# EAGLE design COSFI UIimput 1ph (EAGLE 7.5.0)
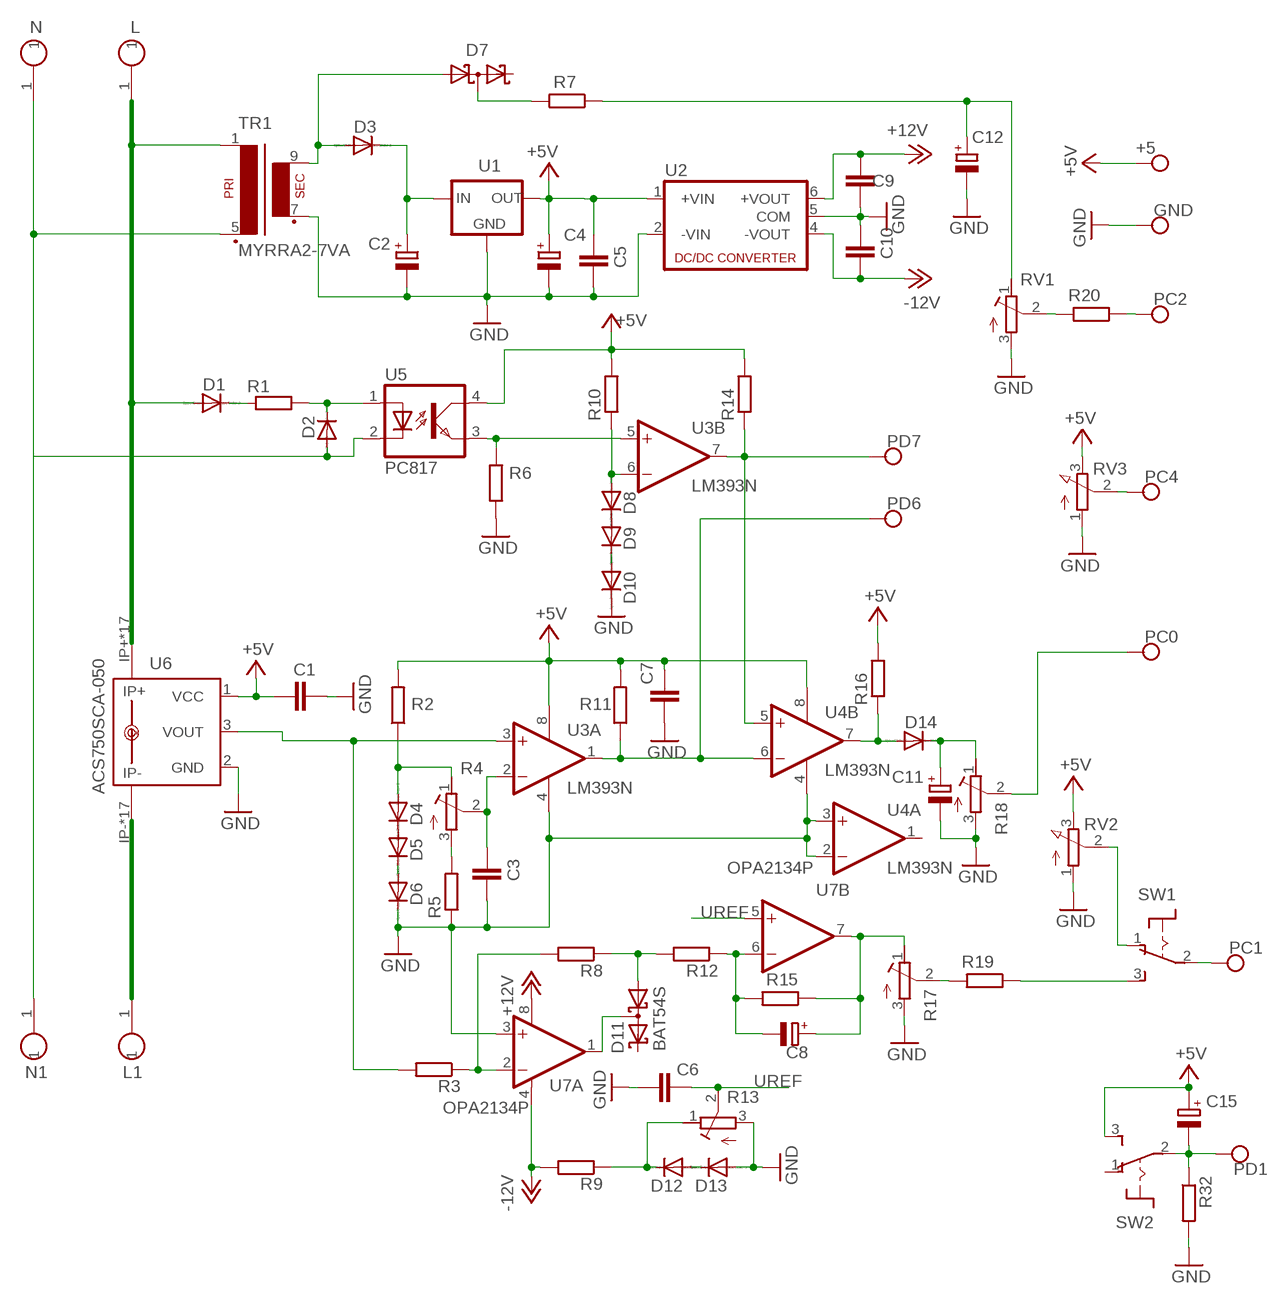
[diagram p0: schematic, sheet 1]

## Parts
+5  CONNWIRE  [CONNWIRE]
C1  C-EUC1206  [C1206]
C2  CPOL-EUE5-8.5  [E5-8,5]
C3  C-EUC1206  [C1206]
C4  CPOL-EUE2-5  [E2-5]
C5  C-EUC1206  [C1206]
C6  C-EUC1206  [C1206]
C7  C-EUC1206  [C1206]
C8  CPOL-EUE2-5  [E2-5]
C9  C-EUC1206  [C1206]
C10  C-EUC1206  [C1206]
C11  CPOL-EUE2-5  [E2-5]
C12  CPOL-EUE3.5-8  [E3,5-8]
C15  CPOL-EUE2-5  [E2-5]
D1  1N4004  [DO41-10]
D2  1N4004  [DO41-10]
D3  1N4004  [DO41-10]
D4  1N4148DO35-7  [DO35-7]
D5  1N4148DO35-7  [DO35-7]
D6  1N4148DO35-7  [DO35-7]
D7  BAT54S  [SOT23]
D8  1N4148DO35-7  [DO35-7]
D9  1N4148DO35-7  [DO35-7]
D10  1N4148DO35-7  [DO35-7]
D11  BAT54S  [SOT23]
D12  1N4148DO35-7  [DO35-7]
D13  1N4148DO35-7  [DO35-7]
D14  1N4148DO35-7  [DO35-7]
GND  CONNWIRE  [CONNWIRE]
L  CONNHOLE  [CONNHOLE4]
L1  CONNHOLE  [CONNHOLE4]
N  CONNHOLE  [CONNHOLE4]
N1  CONNHOLE  [CONNHOLE4]
PC0  CONNWIRE  [CONNWIRE]
PC1  CONNWIRE  [CONNWIRE]
PC2  CONNWIRE  [CONNWIRE]
PC4  CONNWIRE  [CONNWIRE]
PD1  CONNWIRE  [CONNWIRE]
PD6  CONNWIRE  [CONNWIRE]
PD7  CONNWIRE  [CONNWIRE]
R1  R-EU_0617/22  [0617/22]
R2  R-EU_0204/7  [0204/7]
R3  R-EU_0204/7  [0204/7]
R4  R-TRIMM-3386-F  [R-TRIMM-3386F]
R5  R-EU_0204/7  [0204/7]
R6  R-EU_0204/7  [0204/7]
R7  R-EU_0204/7  [0204/7]
R8  R-EU_0204/7  [0204/7]
R9  R-EU_0204/7  [0204/7]
R10  R-EU_0204/7  [0204/7]
R11  R-EU_0204/7  [0204/7]
R12  R-EU_0204/7  [0204/7]
R13  R-TRIMM-3386-F  [R-TRIMM-3386F]
R14  R-EU_0204/7  [0204/7]
R15  R-EU_0204/7  [0204/7]
R16  R-EU_0204/7  [0204/7]
R17  R-TRIMM-3386-F  [R-TRIMM-3386F]
R18  R-TRIMM-3386-F  [R-TRIMM-3386F]
R19  R-EU_0204/7  [0204/7]
R20  R-EU_0204/7  [0204/7]
R32  R-EU_0204/7  [0204/7]
RV1  R-TRIMM-3386-F  [R-TRIMM-3386F]
RV2  PTV09A  PV09A  [PTV09]
RV3  PTV09A  PV09A  [PTV09]
SW1  8MS9P1  [8MS9]
SW2  8MS9P1  [8MS9]
TR1  MYRRA2-7VA  [MYRRA2-7]
U1  78XXL  [78XXL]
U2  NMA  [NMA]
U3  LM393N  [DIL08]
U4  LM393N  [DIL08]
U5  PC817  [DIL04]
U6  ACS750SCA-050  [ACS75050]
U7  OPA2134P  [DIL08]

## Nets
+5V: +5.P$1 C1.2 C4.+ C5.1 C7.2 C15.+ R2.2 R10.2 R11.2 R14.2 R16.2 RV2.3(E) RV3.3(E) SW2.3(S) U1.OUT U2.1(+VIN) U3.8(P:V+) U4.8(P:V+) U5.4(COL) U6.1(VCC)
+12V: C9.1 U2.6(+VOUT) U7.8(A:V+)
-12V: C10.2 R9.2 U2.4(-VOUT) U7.4(A:V-)
GND: C1.1 C2.- C3.2 C4.- C5.2 C6.1 C7.1 C9.2 C10.1 C11.- C12.- D6.C D10.C D13.A GND.P$1 R5.1 R6.1 R13.3(E) R17.3(E) R18.3(E) R32.2 RV1.3(E) RV2.1(A) RV3.1(A) TR1.7(S3) U1.GND U2.2(-VIN) U2.5(COM) U3.4(P:V-) U4.2(A:-IN) U4.3(A:+IN) U4.4(P:V-) U6.2(GND) U7.3(A:+IN)
N$1: D1.C R1.1
N$2: R3.1 R8.2 U7.2(A:-IN)
N$3: D2.C R1.2 U5.1(A)
N$4: D8.C D9.A
N$5: D2.A N1.1 N.1 TR1.5(P2) U5.2(C)
N$6: D1.A L.1 TR1.1 U6.IP+ U6.IP+@2(IP+) U6.IP+@3(IP+) U6.IP+@4(IP+) U6.IP+@5(IP+) U6.IP+@6(IP+) U6.IP+@7(IP+) U6.IP+@8(IP+) U6.IP+@9(IP+) U6.IP+@10(IP+) U6.IP+@11(IP+) U6.IP+@12(IP+) U6.IP+@13(IP+) U6.IP+@14(IP+) U6.IP+@15(IP+) U6.IP+@16(IP+) U6.IP+@17(IP+)
N$7: RV2.2(S) SW1.1(O)
N$8: D9.C D10.A
N$9: D12.A D13.C
N$10: D12.C R9.1 R13.1(A)
N$11: R4.3(E) R5.2
N$12: D4.A R2.1 R4.1(A)
N$13: R6.2 U3.5(B:+IN) U5.3(EMIT)
N$14: R3.2 U3.3(A:+IN) U6.3(VOUT)
N$15: D4.C D5.A
N$16: D8.A R10.1 U3.6(B:-IN)
N$17: D14.A R16.1 U4.7(B:OUT)
N$18: PD7.P$1 R14.1 U3.7(B:OUT) U4.5(B:+IN)
N$19: D5.C D6.A
N$20: PD6.P$1 R11.1 U3.1(A:OUT) U4.6(B:-IN)
N$21: C3.1 R4.2(S) U3.2(A:-IN)
N$22: C11.+ D14.C R18.1(A)
N$23: PC0.P$1 R18.2(S)
N$24: D11.3(C1A2) U7.1(A:OUT)
N$25: PC1.P$1 SW1.2(P)
N$26: PC4.P$1 RV3.2(S)
N$27: R19.1 SW1.3(S)
N$28: PC2.P$1 R20.1
N$29: D3.A D7.1(A1) TR1.9(S4)
N$30: D7.3(C1A2) R7.2
N$31: D11.1(A1) R8.1 R12.2
N$32: C8.- R12.1 R15.2 U7.6(B:-IN)
N$33: C8.+ R15.1 R17.1(A) U7.7(B:OUT)
N$34: C15.- PD1.P$1 R32.1 SW2.2(P)
N$35: R17.2(S) R19.2
N$37: C2.+ D3.C U1.IN
N$38: R20.2 RV1.2(S)
N$40: C12.+ R7.1 RV1.1(A)
N$41: L1.1 U6.IP- U6.IP-@2(IP-) U6.IP-@3(IP-) U6.IP-@4(IP-) U6.IP-@5(IP-) U6.IP-@6(IP-) U6.IP-@7(IP-) U6.IP-@8(IP-) U6.IP-@9(IP-) U6.IP-@10(IP-) U6.IP-@11(IP-) U6.IP-@12(IP-) U6.IP-@13(IP-) U6.IP-@14(IP-) U6.IP-@15(IP-) U6.IP-@16(IP-) U6.IP-@17(IP-)
UREF: C6.2 R13.2(S) U7.5(B:+IN)
Unconnected: D7.2(C2) D11.2(C2) SW2.1(O) U4.1(A:OUT)

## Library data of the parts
+5 GND PC0 PC1 PC2 PC4 PD1 PD6 PD7 = connholes:CONNWIRE
C1 C3 C5-C7 C9 C10 = rcl:C-EU: CAPACITOR, European symbol
C2 C4 C8 C11 C12 C15 = rcl:CPOL-EU: POLARIZED CAPACITOR, European symbol
D1-D3 = diode:1N4004: DIODE
D4-D6 D8-D10 D12-D14 = diode:1N4148: DIODE
D7 D11 = diode:BAT54S: Schottky Diodes Pin connection corrected 2011-05-04 Source: Fairchild .. BAT54.pdf
L L1 N N1 = connholes:CONNHOLE
R1-R3 R5-R12 R14-R16 R19 R20 R32 = rcl:R-EU_: RESISTOR, European symbol
R4 R13 R17 R18 RV1 = rcl:R-TRIMM-3386-F
RV2 RV3 = pot:PV09A
SW1 SW2 = switch:8MS9P1
TR1 = trafo:MYRRA2-7VA
U1 = v-reg:78XXL: VOLTAGE REGULATOR
U2 = dc-dc-converter:NMA: DC-DC CONVERTER; MF: C & D TECHNOLOGIES, INC; MPN: NMA0515SC; OC_FARNELL: 1021434; OC_NEWARK: 61K3064
U3 U4 = linear:LM393: COMPARATOR
U5 = optocoupler:PC817: SHARP OPTO COUPLER; MPN: PC817X4J000F; OC_FARNELL: 9707727; OC_NEWARK: 97K7059
U6 = allegro:ACS750*CA-050: Current Sensor display layer 49 Reference in BRD and place VIAs on circles Source: www.allegromicro.com/datafile/0750-050.pdf; MF: ALLEGRO MICROSYSTEMS, INC.; MPN: ACS750SCA-050; OC_FARNELL: 1457175; OC_NEWARK: 81H6588
U7 = burr-brown:OPA2134: Operational Amplifier; MF: TEXAS INSTRUMENTS; MPN: OPA2134PA; OC_FARNELL: 1097574; OC_NEWARK: 74K3897

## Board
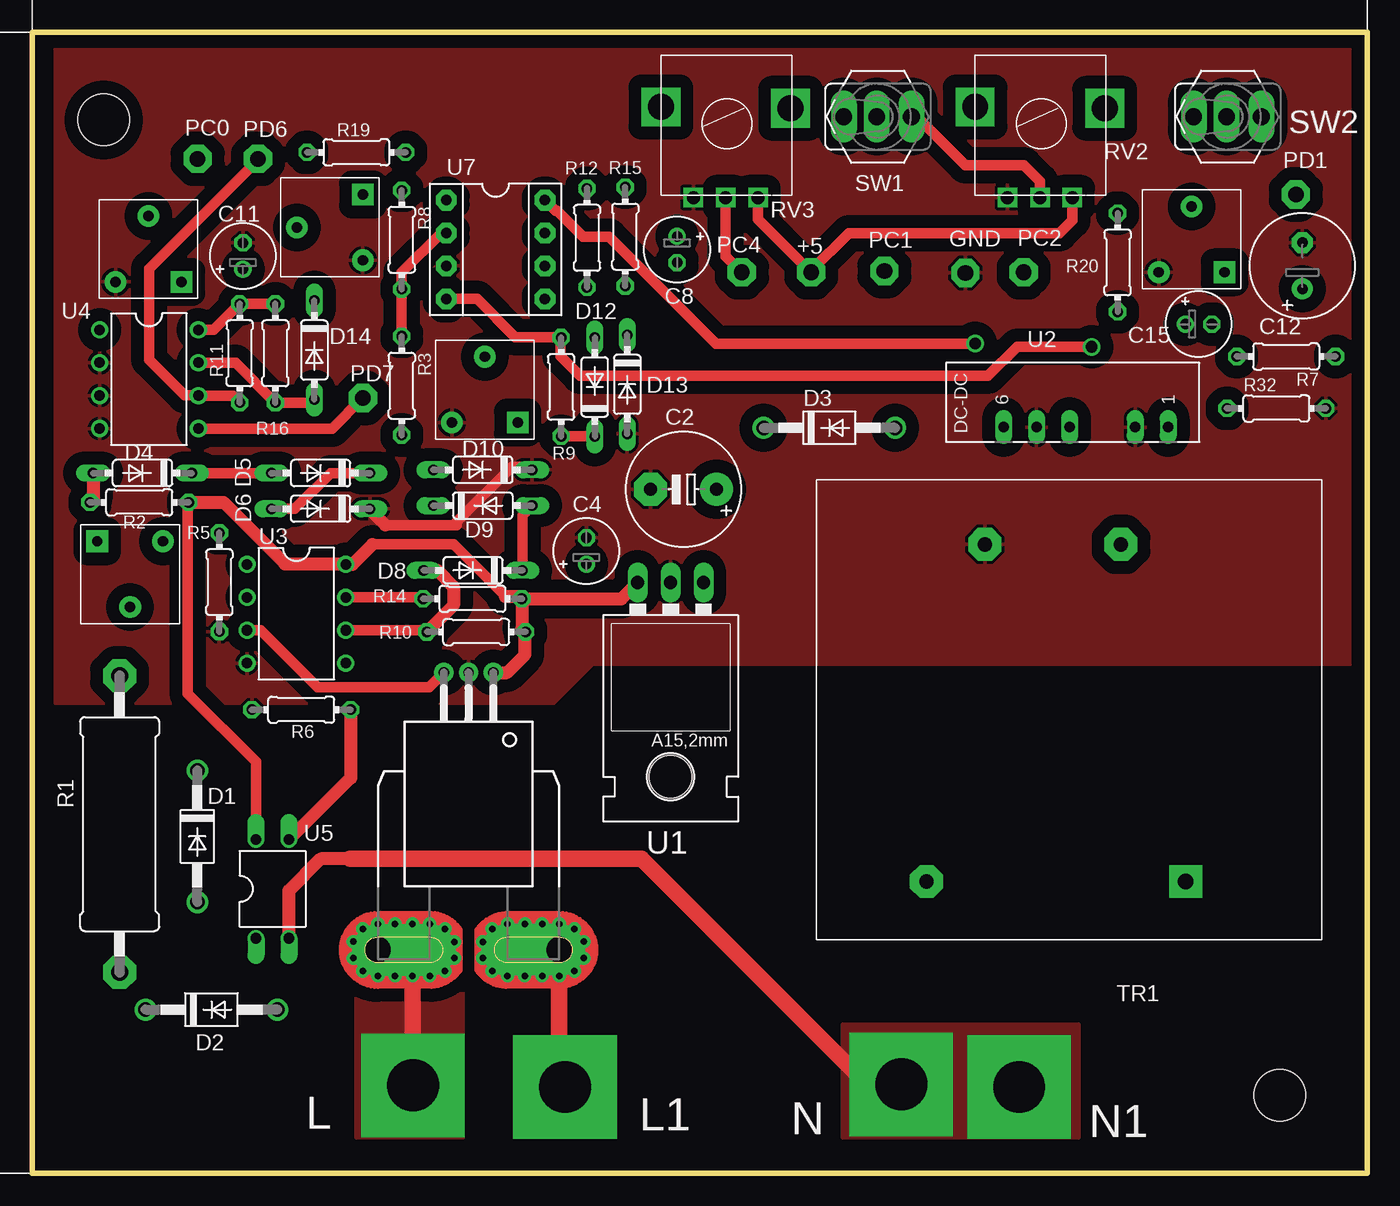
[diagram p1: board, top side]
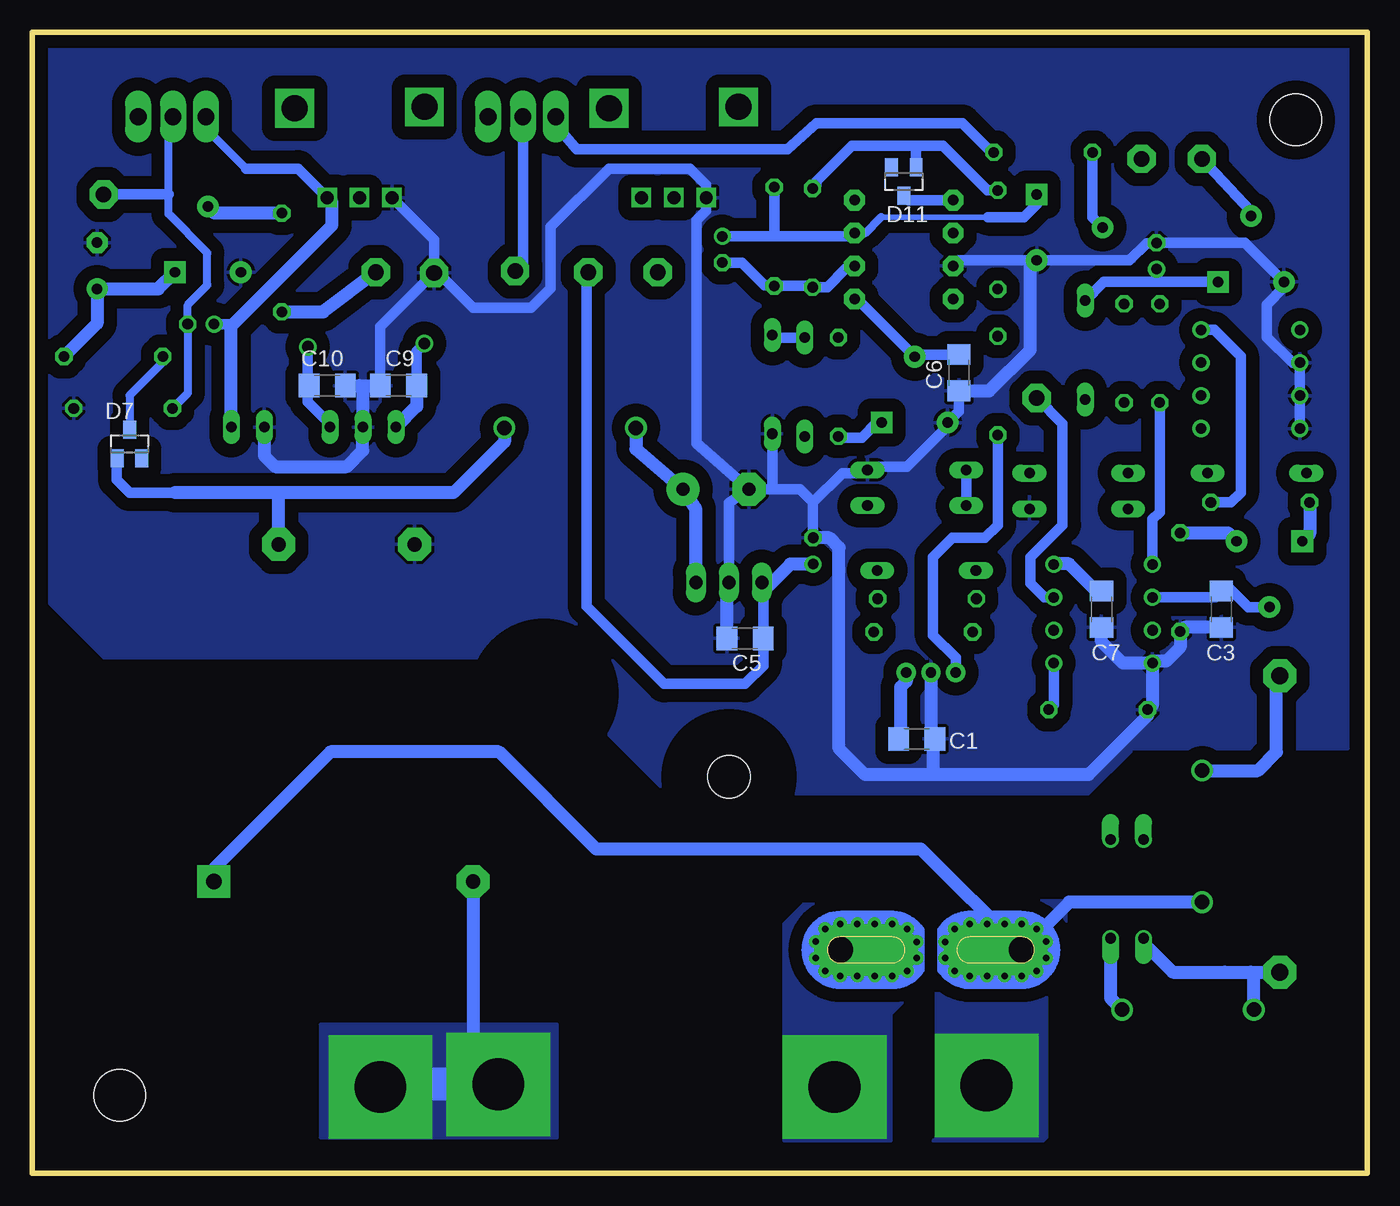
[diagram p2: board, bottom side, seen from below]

Size 103 x 88 mm. Coordinates in mm from the lower left corner, seen from the top.
Outline: 0,0 103,0 103,88 0,88 0,0
Copper layers (1*16): Top 0.035mm / dielectric 1.5mm / Bottom 0.035mm
Design rules "default": minimum track width 10mil, minimum drill 24mil, track to track 8mil, track to pad 8mil, pad to pad 8mil, via to via 8mil, smd to smd 8mil, copper to edge 40mil, drill to drill 8mil, minimum pad ring 10mil, minimum via ring 8mil, stop-mask expansion 4mil, vias tented up to drill 0mil, thermal gap 10mil
Holes 4 mm at 96.25,6 5.5,81.25
bRestrict: area 58.9,32.4 to 68.1,41.6

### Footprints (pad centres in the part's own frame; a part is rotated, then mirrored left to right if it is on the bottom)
CONNWIRE = drill 1.2 pad 2.184 octagon: P$1 0,0
C1206 = smd 1.6 x 1.8: 1 -1.4,0; 2 1.4,0
E5-8,5 = drill 1.016 pad 2.54: + -2.54,0 | drill 1.016 pad 2.54 octagon: - 2.54,0
E2-5 = drill 0.813 pad 1.27: + -1.016,0 | drill 0.813 pad 1.27 octagon: - 1.016,0
E3,5-8 = drill 0.813 pad 1.6: + -1.778,0 | drill 0.813 pad 1.6 octagon: - 1.778,0
DO41-10 = drill 1.118: A 5.08,0; C -5.08,0
DO35-7 = drill 0.813 long: A 3.81,0; C -3.81,0
SOT23 = smd 1 x 1.4: 1 -0.95,-1.1; 2 0.95,-1.1; 3 0,1.1
CONNHOLE4 = drill 4 pad 8 square: 1 0,0
0617/22 = drill 1.3 pad 2.54 octagon: 1 -11.43,0; 2 11.43,0
0204/7 = drill 0.813 octagon: 1 -3.81,0; 2 3.81,0
R-TRIMM-3386F = drill 0.8 pad 1.676 square: 1 0,0 | drill 0.8 pad 1.676: 2 5.08,2.54; 3 0,5.08
PTV09 = drill 1 square: 1 -2.5,0; 2 0,0; 3 2.5,0 | drill 2 square: P$4 -5,7; P$5 5,6.9
8MS9 = drill 1.295 pad 2 long: 1 -3,5.346 | drill 1.3 pad 2 long: 2 -3,2.654; 3 -3,0.114
MYRRA2-7 = drill 1.2 pad 2.54 square: 1 0,0 | drill 1.1 pad 2.54 octagon: 5 20,0; 7 15.5,-26; 9 5,-26
78XXL = drill 1.016 long: GND 0,-3.81; IN -2.54,-3.81; OUT 2.54,-3.81 | hole 3.302: 0,11.176
NMA = drill 0.813 long: 1 0,6.35; 2 0,3.81; 4 0,-1.27; 5 0,-3.81; 6 0,-6.35
DIL08 = drill 0.813 pad 1.27: 1 -3.81,-3.81; 2 -1.27,-3.81; 3 1.27,-3.81; 4 3.81,-3.81; 5 3.81,3.81; 6 1.27,3.81; 7 -1.27,3.81; 8 -3.81,3.81
DIL04 = drill 0.813 offset: 1 -1.27,-3.81; 2 1.27,-3.81; 3 1.27,3.81; 4 -1.27,3.81
ACS75050 = drill 0.8 pad 1.5: 1 -1.91,-21.4; 2 0,-21.4; 3 1.91,-21.4 | drill 2 pad 4 offset: IP+ 7,0; IP- -7,0 | drill 0.5 pad 0.9: IP+@2 8.89,-0.635; IP+@3 8.89,0.635; IP+@4 8.175,1.625; IP+@5 7,2; IP+@6 5.675,2; IP+@7 4.325,2; IP+@8 3,2; IP+@9 1.825,1.625; IP+@10 1.1,0.625; IP+@11 1.1,-0.625; IP+@12 1.825,-1.625; IP+@13 3,-2; IP+@14 4.325,-2; IP+@15 5.675,-2; IP+@16 7,-2; IP+@17 8.175,-1.625; IP-@2 -8.89,-0.635; IP-@3 -8.89,0.635; IP-@4 -8.175,1.625; IP-@5 -7,2; IP-@6 -5.675,2; IP-@7 -4.325,2; IP-@8 -3,2; IP-@9 -1.825,1.625; IP-@10 -1.1,0.625; IP-@11 -1.1,-0.625; IP-@12 -1.825,-1.625; IP-@13 -3,-2; IP-@14 -4.35,-2; IP-@15 -5.675,-2; IP-@16 -7,-2; IP-@17 -8.175,-1.625
DIL08' = drill 0.813 pad 1.6 octagon: 1 -3.81,-3.81; 2 -1.27,-3.81; 3 1.27,-3.81; 4 3.81,-3.81; 5 3.81,3.81; 6 1.27,3.81; 7 -1.27,3.81; 8 -3.81,3.81

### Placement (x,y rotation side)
+5  60.1,69.5 270 top
C1  34.75,33.5 180 bottom
C2  50.25,52.75 180 top
C3  11.25,43.5 270 bottom
C4  42.75,48 90 top
C5  48,41.25 180 bottom
C6  31.5,61.75 90 bottom
C7  20.5,43.5 90 bottom
C8  49.75,71.25 270 top
C9  74.75,60.75 180 bottom
C10  80.25,60.75 180 bottom
C11  16.25,70.75 90 top
C12  98,70 90 top
C15  90,65.5 0 top
D1  12.73,25.98 270 top
D2  13.82,12.61 0 top
D3  61.5,57.5 0 top
D4  8.5,54 180 top
D5  22.25,54 180 top
D6  22.25,51.25 180 top
D7  95.5,56.25 0 bottom
D8  34,46.5 180 top
D9  34.75,51.5 0 top
D10  34.75,54.25 180 top
D11  35.75,76.5 180 bottom
D12  43.4,60.65 90 top
D13  45.9,60.85 270 top
D14  21.75,63.5 270 top
GND  72,69.45 0 top
L  29.37,6.77 0 top
L1  41.1,6.65 0 top
N  67.05,6.85 0 top
N1  76.15,6.65 0 top
PC0  12.75,78.25 0 top
PC1  65.75,69.6 0 top
PC2  76.5,69.5 0 top
PC4  54.75,69.5 90 top
PD1  97.5,75.5 0 top
PD6  17.4,78.25 270 top
PD7  25.5,59.8 0 top
R1  6.73,26.93 270 top
R2  8.25,51.75 0 top
R3  28.5,60.75 270 top
R4  5,48.75 270 top
R5  14.43,45.59 90 top
R6  20.75,35.75 0 top
R7  96.75,63 180 top
R8  28.5,72 270 top
R9  40.8,60.65 90 top
R10  34.25,41.75 0 top
R11  16,63.25 90 top
R12  42.8,72.15 90 top
R13  37.45,57.9 90 top
R14  33.96,44.31 0 top
R15  45.75,72.25 270 top
R16  18.75,63.25 90 top
R17  25.5,75.5 180 top
R18  11.5,68.75 90 top
R19  25,78.75 180 top
R20  83.75,70.25 90 top
R32  96,59 0 top
RV1  92,69.5 90 top
RV2  77.75,75.25 0 top
RV3  53.5,75.25 0 top
SW1  62.5,78.5 270 top
SW2  89.5,78.5 270 top
TR1  89,22.5 180 top
U1  49.25,41.75 180 top
U2  81.3,57.55 270 top
U3  20.37,43.15 270 top
U4  9,61.25 270 top
U5  18.53,21.93 0 top
U6  33.66,17.22 180 top
U7  OPA2134P  [DIL08']  35.75,71.25 270 top

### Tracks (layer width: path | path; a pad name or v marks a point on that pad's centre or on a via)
+5V
  Top 0.813: U5.4 17.26,31.74 12,37 12,51.69 R2.2 | RV2.3 80.25,73.5 79.25,72.5 63,72.5 60.1,69.6 +5.P$1 56,73.6 RV3.3 | R16.2 R11.2 14,65.06 U4.8 | 26.25,48.5 32.5,48.5 36.5,44.5
  Top 1.016: R2.2 14.75,51.75 19.5,47 24.14,47 U3.8 24.71,46.96 26.25,48.5 | 36.5,44.5 37.58,44.5 R14.2 | R14.2 37.77,42.04 R10.2 38,41.69 38,40 36.62,38.62 U6.1 | R14.2 45.46,44.31 U1.OUT
  Bottom 0.61: SW2.3 89.61,80.61 86.5,77.5
  Bottom 0.813: +5.P$1 60.25,69.35 60.25,43.75 54.25,37.75 48,37.75 46.6,39.15 C5.1 46.6,45.45 | U4.8 11.81,65.06 9.75,63 9.75,52.5 10.5,51.75 R2.2 | 86.5,77.5 82.5,77.5 RV2.3 | C15.+ 87.8,65.5 87.65,65.35
  Bottom 1.016: C7.2 20.9,44.9 23,47 24.14,47 U3.8 | 46.6,45.45 U1.OUT 46.33,45.17 44.52,46.98 C4.+ | U6.1 35.57,37.93 36,37.5 36,33.65 C1.2 | U2.1 87.65,65.35 79.88,73.12 79.88,74.88 RV2.3
+12V  (via drill 0.9)
  Top 0.813: v72.75,64 52.75,64 44.5,72.25 42.5,72.25 40.5,74.25 40.37,74.25 U7.8
  Bottom 0.813: C9.1 73.35,63.4 v72.75,64
  Bottom 1.016: C9.1 73.35,59.15 U2.6
-12V  (via drill 0.9)
  Top 0.813: v81.75,63.75 76,63.75 73.75,61.5 42.25,61.5 40.75,63 40.75,64.41 R9.2 40.76,64.5 37.25,64.5 34.31,67.44 U7.4
  Bottom 0.813: v81.75,63.75 81.75,60.65 81.75,59.5 80.03,57.78
  Bottom 1.016: U2.4 80.03,57.78 | 81.75,60.65 C10.2
GND
  Top 0.813: 27.25,50 32.75,50 32.75,50.25 37,54.5 38.31,54.5 D10.C
  Top 1.016: D6.C 26.06,51.19 27.25,50
  Bottom 0.813: C6.1 31.5,58.77 R13.3 32.37,57.63 35.5,54.5 38.31,54.5 D10.C 38.81,54 40.5,54 42.75,51.75 | C4.- 42.75,51.75 | C2.- 45.75,52.75 | 45.75,52.75 43.75,52.75 42.75,51.75 | U1.GND 49.25,51.71 C2.- | GND.P$1 72,72 RV2.1 | GND.P$1 71.7,69.45 69,66.75 64.5,66.75 63,68.25 63,73 58.5,77.5 52.25,77.5 51,76.25 RV3.1 51,74.25 51.75,73.5 51.75,56.29 C2.- | C9.2 76.15,65.3 GND.P$1 | D13.A 45.9,52.9 45.75,52.75 | U7.3 31.5,70.42 R17.3 18.33,70.42 17,71.75 16.27,71.75 C11.- 9.44,71.77 R18.3 6.42,68.33 7.75,67 7.75,64.5 5.75,62.5 5.21,62.5 U4.2 U4.3 U4.4
  Bottom 1.016: U3.4 16.56,36.13 R6.1 16.94,35.31 21.5,30.75 33.5,30.75 | C3.2 14.11,42.1 R5.1 14.43,40.57 15.5,39.5 16.4,39.5 U3.4 | U3.4 18.84,39.34 20.5,41 C7.1 | C5.2 49.4,45.41 U1.GND | C1.1 33.66,33.81 U6.2 33.66,33.66 33.5,33.5 33.5,30.75 | C10.1 77.75,60.75 | 77.75,60.75 C9.2 | 77.75,60.75 77.49,60.49 U2.5 77.5,55.75 78.75,54.5 84.25,54.5 85.11,55.36 U2.2 | 33.5,30.75 38.75,30.75 40.75,32.75 40.75,48.25 41.5,49 42.73,49 C4.- | C6.1 29.15,60.35 26,63.5 26,69.92 R17.3
  pour Bottom (isolate 1.016): 2.75,32.75 18.25,32.75 18.25,32.5 21.5,29.25 54,29.25 64.5,39.75 97.5,39.75 102.25,44.5 103,45.25 103,87 102.25,87.75 1.75,87.75 1.5,87.5 1.5,32.75
  pour Top (isolate 1): 2,87.5 102.5,87.5 102.5,39.5 102.75,39.25 43.25,39.25 40.25,36.25 2.25,36.25 1.75,36.25 1.75,87.5
N$1
  Bottom 1.016: D1.C 8.44,31.06 7,32.5 7,38.09 R1.1
N$2
  Top 0.813: R3.1 R8.2 28.5,69.5 31.52,72.52 U7.2
N$3
  Bottom 1.016: U5.1 17.26,17.76 15,15.5 11,15.5 | 11,15.5 9,15.5 | 9,15.5 R1.2 | 10.99,15.49 11,15.5 | D2.C 8.74,15.24 9,15.5
N$4
  Top 0.813: D8.C 37.81,50.75 D9.A
N$5
  Top 1.016: 24.5,24.25 22.25,24.25 19.8,21.8 U5.2
  Top 1.27: N.1 64.4,6.85 47,24.25 24.5,24.25
  Bottom 1.016: U5.2 19.8,13.51 D2.A | TR1.5 69,9.35 66.5,6.85
  Bottom 2.54: N.1 75.95,6.85 N1.1
  pour Bottom (isolate 1.016, no thermals): 62.5,11.5 80.75,11.5 80.75,2.75 62.5,2.75
  pour Top (isolate 1.016, no thermals): 62.5,11.5 80.75,11.5 80.75,2.75 62.5,2.75
N$6
  Top 1.27: U6.IP+@7 29.34,6.8 L.1
  Bottom 1.016: D1.A 22.98,20.9 U6.IP+ 34.44,25 59.5,25 67,32.5 80,32.5 89.5,23 TR1.1
  pour Top (isolate 1.016, no thermals): 23.75,20.75 32.25,20.75 33.25,19.75 33.25,2.75 25,2.75 25,14 23.5,15.5 23.5,20.5
  pour Bottom (isolate 1.016, no thermals): 23.5,21 31.75,21 33.25,19.5 33.25,2.75 33.5,2.5 25,2.5 24.75,2.75 24.75,13.75 23.25,15.25 23.25,21
N$7
  Top 0.813: SW1.1 68.25,81.5 72,77.75 76.5,77.75 77.75,76.5 RV2.2
N$8
  Bottom 0.813: D10.A D9.C
N$9
  Bottom 0.813: D12.A 45.7,64.46 D13.C
N$10
  Top 0.813: R9.1 D12.C
  Bottom 0.813: R13.1 37.85,57.9 39,56.75 40.71,56.75 R9.1
N$11
  Bottom 1.016: R5.2 10.73,49.4 R4.3
N$12
  Top 1.016: D4.A 4.69,52 R2.1
  Bottom 1.016: R2.1 4.44,49.31 R4.1
N$13
  Top 1.016: R6.2 24.56,30.5 U5.3
  Bottom 0.813: U3.5 24.18,36.13 R6.2
N$14
  Top 0.813: U3.3 17.62,41.88 22,37.5 30.63,37.5 U6.3
  Bottom 0.813: U6.3 31.75,39.75 33.5,41.5 33.5,47.5 32,49 29.5,49 28.5,50 R3.2
N$15
  Top 0.813: D5.A D4.C
N$16
  Top 0.813: U3.6 30.31,41.88 R10.1
  Top 1.016: D8.A 31.25,46.5 32.5,45.25 32.5,43.81 R10.1
  Bottom 0.813: 30.31,41.88 R10.1
N$17
  Top 0.813: U4.7 15.67,62.52 R16.1 21.5,59.44 D14.A
N$18
  Top 0.813: U3.7 30.04,44.42 R14.1 | U4.5 23.14,57.44 PD7.P$1
  Bottom 0.813: U3.7 24.92,44.42 26,45.5 26,47.5 23.5,50 23.5,57.8 PD7.P$1
N$19
  Top 0.813: D6.A 20.25,51.25 23,54 D5.C
N$20
  Top 0.813: R11.1 15.46,59.98 U4.6 12.79,60 11.75,60 9,62.75 9,69.75 17.4,78.15 PD6.P$1
  Bottom 0.813: U3.1 16.56,50.44 16,51 R11.1
N$21
  Bottom 0.813: U3.2 11.73,44.42 C3.1 11.15,45 10.5,45 9.17,43.67 R4.2
N$22
  Bottom 0.813: R18.1 16.5,68.75 | 16.5,68.75 20.31,68.75 D14.C | C11.+ 16.25,69 16.5,68.75
N$23
  Bottom 0.813: R18.2 8.96,74.21 PC0.P$1
N$24
  Bottom 0.813: U7.1 35.41,75.06 D11.3
N$25
  Bottom 0.813: SW1.2 65.15,70.2 PC1.P$1
N$26
  Top 0.813: RV3.2 53.5,70.75 PC4.P$1
N$27
  Bottom 0.813: R19.1 29,78.75 31.25,81 42.5,81 44.75,79 61,79 62.5,80.75 62.5,81.39 SW1.3
N$28
  Bottom 1.016: R20.1 80.56,66.44 PC2.P$1
N$29
  Bottom 0.813: 92,52.5 95.5,52.5 96.5,53.5 96.5,55.1 D7.1
  Bottom 1.016: D3.A 66.58,56.42 70.5,52.5 84,52.5 | 84,52.5 92,52.5 | TR1.9 84,52.5
N$30
  Bottom 0.61: 93,62.94 93,62.5 95.5,60 D7.3
  Bottom 1.016: 93,62.94 R7.2
N$31
  Bottom 0.813: R8.1 29.31,75.81 32.75,79.25 34.75,79.25 | 34.75,79.25 39.75,79.25 42.5,76.5 42.5,76.26 R12.2 | D11.1 34.8,79.2 34.75,79.25
N$32
  Bottom 0.813: C8.- 48.23,70.23 46.5,68.5 45.81,68.5 R15.2 42.9,68.44 R12.1 41.66,68.34 40.25,69.75 39.79,69.75 U7.6
N$33
  Bottom 0.406: 37.5,73.75 29.25,73.75
  Bottom 0.61: U7.7 38.73,72.52 37.5,73.75
  Bottom 0.813: C8.+ 45.75,72.27 | 45.75,72.27 39.81,72.27 U7.7 | R15.1 45.75,72.27 | 29.25,73.75 26.5,73.75 25.5,74.75 R17.1
N$34
  Bottom 0.61: SW2.2 92.5,81.15 92.5,75.5 92.5,74 89.5,71 89.5,68.5 91.02,66.98 C15.- 91.02,60.17 R32.1
  Bottom 0.813: PD1.P$1 92.5,75.5
N$35
  Bottom 0.813: R19.2 21.19,73.73 R17.2
N$37
  Bottom 1.016: U1.IN 51.79,51.25 C2.+ 56.42,55.88 D3.C
N$38
  Bottom 1.016: R20.2 88.94,74.06 RV1.2
N$40
  Bottom 1.016: RV1.1 93.28,68.22 C12.+ 98,65.56 R7.1
N$41
  Top 1.27: U6.IP-@5 40.66,7.09 L1.1
  pour Bottom (isolate 1.016, no thermals): 34.25,20.75 43.5,20.75 44.5,19.75 45,19.25 45,2.5 36.75,2.5 36.75,12.25 34.25,14.75
UREF
  Bottom 0.813: C6.2 34.74,63.15 R13.2 39.37,67.44 U7.5

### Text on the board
tNames: N1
